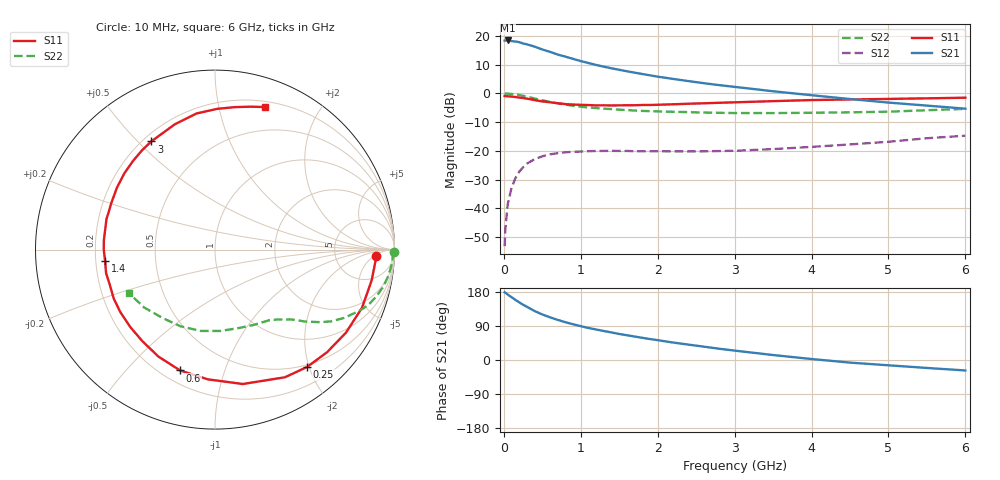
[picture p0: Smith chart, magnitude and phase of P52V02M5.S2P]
! SIEMENS Small Signal Semiconductors
! BFP183
! Si NPN RF Bipolar Junction Transistor in SOT143
! VCE = 2 V  IC = 2.5 mA
! Common Emitter S-Parameters:  March  1996
# GHz  S  MA  R  50
!  f  S11  S21  S12  S22
! GHz  MAG  ANG  MAG  ANG  MAG  ANG  MAG  ANG
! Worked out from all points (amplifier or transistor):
!   36 points, 10 MHz to 6 GHz, reference 50 ohm
!   highest |S21| = 18.4 dB at 50 MHz (marker M1)
!   |S21| within 3 dB of that: start of sweep to 486.1 MHz
!   unconditionally stable (mu >= 1): 1.939 GHz to 5.838 GHz
!   at 250 MHz: K = 0.14, MSG = 21.5 dB, |S12| = -25.7 dB
!   at 1.4 GHz: K = 0.74, MSG = 14.4 dB, |S12| = -20.0 dB
!   at 6 GHz: K = 0.97, MSG = 4.7 dB, |S12| = -14.7 dB
!   S11 on the Smith chart (normalised r, x): 10 MHz: 17, -6; 250 MHz: 0.46, -1.97; 600 MHz: 0.27, -0.72; 1.4 GHz: 0.24, -0.05; 3 GHz: 0.23, +0.55; 6 GHz: 0.25, +1.38
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0.01  0.8998 -2.3  8.262 178.8  0.0022 89.7  0.9978 -0.8
0.02  0.8959 -4.4  8.294 177.7  0.0044 84.4  0.991 -1.7
0.05  0.8896 -11.1  8.331 172.8  0.0117 85.4  0.9899 -4.3
0.15  0.864 -32.4  7.984 158.7  0.0334 72.3  0.9593 -12.6
0.2  0.8467 -42.4  7.787 152.1  0.0434 66.8  0.935 -16.3
0.25  0.8313 -51.9  7.387 145.9  0.0518 61.7  0.9081 -19.9
0.3  0.811 -61.3  7.135 140.4  0.0601 57.0  0.8769 -22.7
0.4  0.7647 -78.3  6.507 129.2  0.0716 49.2  0.8152 -27.8
0.5  0.7241 -93.1  5.805 120.2  0.0805 42.1  0.7591 -31.8
0.6  0.7009 -106.1  5.272 112.7  0.0871 36.8  0.7121 -34.6
0.7  0.6741 -117.9  4.74 105.9  0.0911 32.5  0.6714 -36.8
0.8  0.6512 -128.4  4.356 99.7  0.0944 28.8  0.6389 -38.8
0.9  0.6395 -137.6  3.987 94.4  0.0964 25.9  0.6091 -40.4
1.1  0.6267 -154.2  3.379 84.5  0.0987 21.5  0.5676 -43.2
1.4  0.6158 -174.1  2.73 72.7  0.1001 16.8  0.5325 -47.1
1.8  0.6281 164.3  2.172 58.5  0.0986 14.8  0.4956 -52.6
2.2  0.6464 147.6  1.785 46.1  0.0981 14.7  0.4779 -59.1
3  0.6995 120.5  1.299 24.8  0.1004 18.2  0.4551 -75.0
3.5  0.7331 107.8  1.089 13.1  0.1074 21.1  0.4543 -86.4
4.5  0.7846 89.0  0.798 -6.9  0.1295 23.8  0.4685 -114.2
5.5  0.8203 76.1  0.613 -21.0  0.1659 22.3  0.5096 -140.7
6  0.841 70.8  0.542 -27.6  0.1835 18.8  0.5376 -153.1
